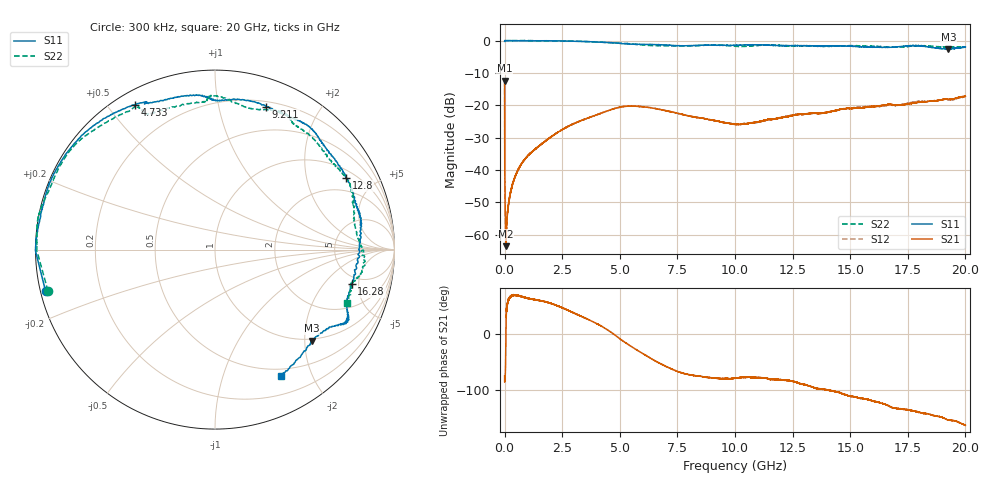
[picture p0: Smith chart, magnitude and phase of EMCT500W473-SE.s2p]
!EMCT500W473
!Johanson Technology Inc.
!www.johansontechnology.com
!Test Board Conditions:
!Substrate Type  RO4350B
!Substrate Thickness  10 mil
!Substrate Dk  3.66
!TL Type: GCPW
!TL Trace Width  22 mil
!TL Gap  14 mil
!PART MODE SINGLE ENDED (AKA BYPASS)
!DUT TOPOLOGY	SERIES-SHUNT
# MHz S  dB  R 50
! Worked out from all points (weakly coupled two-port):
!   20001 points, 300 kHz to 20 GHz, reference 50 ohm
!   highest |S21| = -12.44 dB at 300 kHz (marker M1); lowest = -63.5 dB at 55.3 MHz (marker M2)
!   lowest |S11| = -2.6 dB at 19.26 GHz (marker M3), VSWR 6.67, Z = 48.2 - j108 ohm
!   |S11| at or under -10 dB: nowhere
!   |S22| runs from -2.2 to 0.0 dB; largest |S21 - S12| = 0.0056
!   S11 on the Smith chart (normalised r, x): 300 kHz: 0.01, -0.12; 4.733 GHz: 0.06, +0.59; 9.211 GHz: 0.25, +1.39; 12.8 GHz: 1.32, +3.44; 16.28 GHz: 4.11, -4.11; 20 GHz: 0.41, -1.57
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0.3  -0.25 -166.3  -12.44 -75.5  -12.39 -75.5  -0.37 -166.1
55.299  -0.01 179.4  -63.54 -6.1  -63.03 -13.3  -0.06 179.5
101.298  -0.01 178.8  -54.80 49.1  -55.03 51.0  -0.08 178.9
121.298  -0.01 178.6  -53.48 56.7  -53.51 56.2  -0.07 178.8
231.297  -0.03 177.4  -47.82 67.6  -47.94 67.5  -0.07 177.4
373.294  -0.02 175.9  -43.90 71.2  -43.70 70.4  -0.05 175.6
853.287  -0.08 170.7  -36.90 67.5  -36.96 67.1  0.02 169.9
2093.269  -0.08 153.7  -29.37 54.9  -29.32 54.7  -0.16 157.7
3334.25  -0.27 135.2  -24.70 32.4  -24.72 32.5  -0.23 142.8
4733.229  -0.71 118.8  -21.09 0.5  -21.11 0.4  -0.72 125.8
6667.2  -1.27 95.8  -21.20 -51.0  -21.17 -51.4  -1.58 112.6
7881.182  -1.59 88.3  -23.11 -71.9  -23.08 -71.4  -1.66 95.5
9211.162  -1.46 70.4  -24.90 -79.7  -24.94 -79.1  -1.34 89.7
10000.15  -1.46 61.4  -25.91 -79.4  -25.75 -79.2  -1.76 79.9
12803.11  -1.59 28.7  -22.77 -88.8  -22.72 -89.3  -1.66 53.2
13334.1  -1.65 20.9  -22.50 -94.9  -22.46 -95.4  -1.72 45.9
15045.07  -1.72 6.5  -21.03 -112.6  -20.86 -111.4  -1.57 27.1
16281.06  -2.09 -14.1  -20.18 -123.5  -20.39 -124.8  -1.88 16.1
16667.05  -2.10 -19.6  -19.77 -129.6  -19.97 -128.6  -2.02 12.5
17907.03  -1.63 -29.3  -19.14 -139.9  -18.93 -140.3  -1.64 -3.9
19260.01  -2.62 -43.3  -18.23 -155.4  -18.30 -156.0  -2.15 -13.9
20000  -1.99 -62.6  -17.22 -164.9  -17.36 -163.2  -1.97 -22.2
